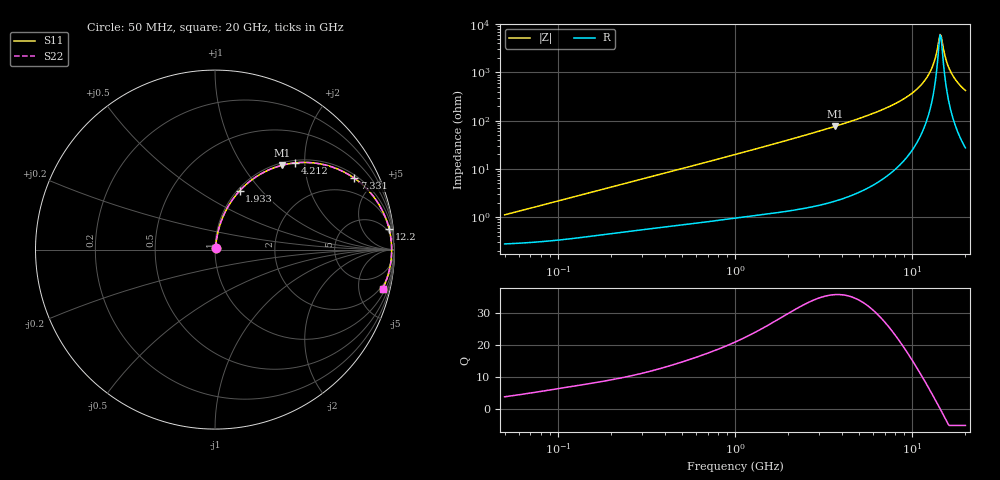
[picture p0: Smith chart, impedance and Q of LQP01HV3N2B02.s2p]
!Murata Part Number: LQP01HV3N2B02
!These Parameters are Measured in Series Mode Connection
!  o--[Z]--o
!Port1  Port2
!  o-------o
!Freq. Start=50[MHz] Stop=20[GHz], 401[Steps]
# Hz S RI R 50
!Freq.(Hz) S11(Real) S11(Imag) S21(Real) S21(Imag) S12(Real) S12(Imag) S22(Real) S22(Imag)
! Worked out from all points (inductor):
!   401 points, 50 MHz to 20 GHz, reference 50 ohm
!   read as one part in series: L = 3.43 nH near 51.52 MHz
!   highest Q = 35.6 at 3.681 GHz (marker M1), where L = 3.31 nH
!   self-resonance near 14.39 GHz
!   S11 on the Smith chart (normalised r, x): 50 MHz: 1.01, +0.02; 1.933 GHz: 1.03, +0.77; 4.212 GHz: 1.05, +1.79; 7.331 GHz: 1.15, +3.82; 12.2 GHz: 3, +16; 20 GHz: 1.55, -8.44
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5e7  0.0029 0.0107  0.9971 -0.0107  0.9971 -0.0107  0.0029 0.0107
1.364002e8  0.00461 0.0286  0.9954 -0.0286  0.9954 -0.0286  0.00461 0.0286
3.721004e8  0.0116 0.0742  0.9884 -0.0742  0.9884 -0.0742  0.0116 0.0742
1e9  0.0462 0.1874  0.9538 -0.1874  0.9538 -0.1874  0.0462 0.1874
1.932977e9  0.137 0.3272  0.863 -0.3272  0.863 -0.3272  0.137 0.3272
2.728004e9  0.2391 0.412  0.7609 -0.412  0.7609 -0.412  0.2391 0.412
3.680849e9  0.3724 0.4696  0.6276 -0.4696  0.6276 -0.4696  0.3724 0.4696
4.212059e9  0.4456 0.4831  0.5544 -0.4831  0.5544 -0.4831  0.4456 0.4831
5.598765e9  0.6167 0.4709  0.3833 -0.4709  0.3833 -0.4709  0.6167 0.4709
7.331367e9  0.7767 0.3975  0.2233 -0.3975  0.2233 -0.3975  0.7767 0.3975
7.442007e9  0.7849 0.3916  0.2151 -0.3916  0.2151 -0.3916  0.7849 0.3916
1.004137e10  0.92 0.2402  0.08 -0.2402  0.08 -0.2402  0.92 0.2402
1.115139e10  0.9511 0.175  0.0489 -0.175  0.0489 -0.175  0.9511 0.175
1.220001e10  0.9698 0.1159  0.0302 -0.1159  0.0302 -0.1159  0.9698 0.1159
1.314879e10  0.9796 0.0652  0.0204 -0.0652  0.0204 -0.0652  0.9796 0.0652
1.417136e10  0.984 0.0136  0.016 -0.0136  0.016 -0.0136  0.984 0.0136
1.438523e10  0.9842 0.00325  0.0158 -0.00325  0.0158 -0.00325  0.9842 0.00325
1.482269e10  0.984 -0.0175  0.016 0.0175  0.016 0.0175  0.984 -0.0175
1.573793e10  0.981 -0.0588  0.019 0.0588  0.019 0.0588  0.981 -0.0588
1.670968e10  0.9744 -0.0997  0.0256 0.0997  0.0256 0.0997  0.9744 -0.0997
1.828096e10  0.9582 -0.1597  0.0418 0.1597  0.0418 0.1597  0.9582 -0.1597
2e10  0.9345 -0.2172  0.0655 0.2172  0.0655 0.2172  0.9345 -0.2172
